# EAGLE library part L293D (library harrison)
L293D Quad Half-H Motor Driver
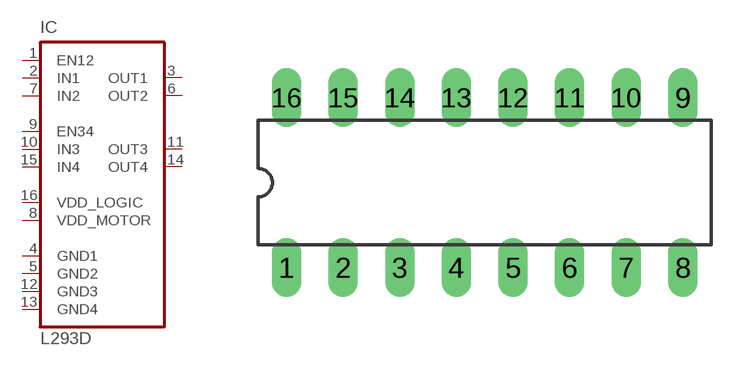
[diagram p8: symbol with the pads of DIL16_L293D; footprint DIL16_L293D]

Designator prefix IC

## L293D  [DIL16_L293D]
1  EN12  in
2  IN1  in
3  OUT1  out
4  GND1  pwr
5  GND2  pwr
6  OUT2  out
7  IN2  in
8  VDD_MOTOR  pwr
9  EN34  in
10  IN3  in
11  OUT3  out
12  GND3  pwr
13  GND4  pwr
14  OUT4  out
15  IN4  in
16  VDD_LOGIC  pwr

## Footprint DIL16_L293D (pad centres in mm)
drill 0.813 long: 1 -8.89,-3.81; 2 -6.35,-3.81; 3 -3.81,-3.81; 4 -1.27,-3.81; 5 1.27,-3.81; 6 3.81,-3.81; 7 6.35,-3.81; 8 8.89,-3.81; 9 8.89,3.81; 10 6.35,3.81; 11 3.81,3.81; 12 1.27,3.81; 13 -1.27,3.81; 14 -3.81,3.81; 15 -6.35,3.81; 16 -8.89,3.81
